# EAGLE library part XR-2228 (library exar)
Operational MULTIPLIER
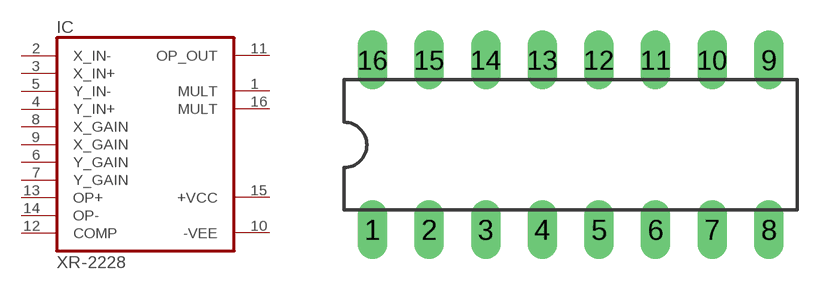
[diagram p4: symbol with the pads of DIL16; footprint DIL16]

Designator prefix IC

## XR-2228 (OC_FARNELL: unknown; OC_NEWARK: unknown)  [DIL16]
1  MULT  out
2  X_IN-  in
3  X_IN+  in
4  Y_IN+  in
5  Y_IN-  in
6  Y_GAIN  in
7  Y_GAIN  in
8  X_GAIN  in
9  X_GAIN  in
10  -VEE  pwr
11  OP_OUT  out
12  COMP  in
13  OP+  in
14  OP-  in
15  +VCC  pwr
16  MULT  out

## Footprint DIL16 (pad centres in mm)
Dual In Line Package
drill 0.813 long: 1 -8.89,-3.81; 2 -6.35,-3.81; 3 -3.81,-3.81; 4 -1.27,-3.81; 5 1.27,-3.81; 6 3.81,-3.81; 7 6.35,-3.81; 8 8.89,-3.81; 9 8.89,3.81; 10 6.35,3.81; 11 3.81,3.81; 12 1.27,3.81; 13 -1.27,3.81; 14 -3.81,3.81; 15 -6.35,3.81; 16 -8.89,3.81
